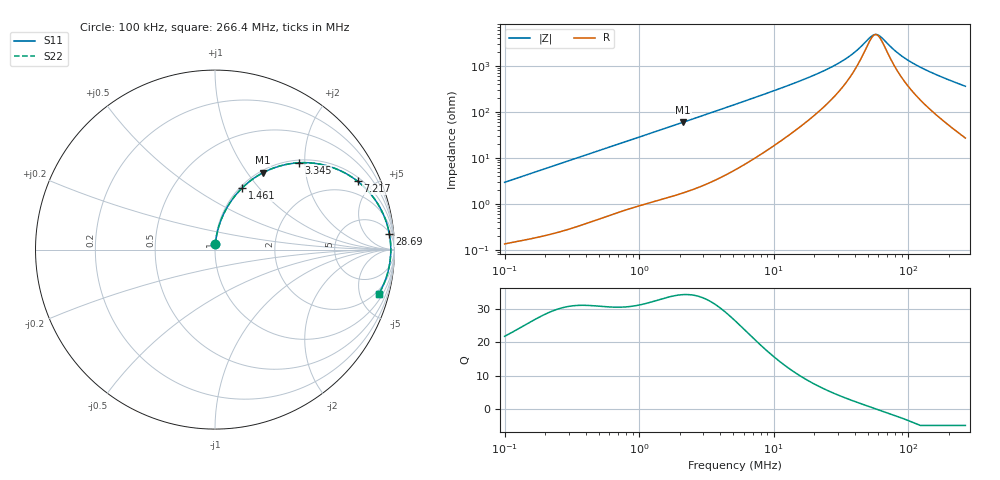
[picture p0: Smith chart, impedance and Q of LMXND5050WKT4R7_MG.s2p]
! LMXND5050WKT4R7_MG  S-PARAMETER MODEL  ( General Type )
! Model Generated by TAIYO YUDEN Corporation (http://www.ty-top.com)
! Version 1.0
! TAIYO YUDEN Control No. 191023NI43SB-FBB
! Copyright(c) 2019 TAIYO YUDEN CO.,LTD. All Rights Reserved.
! Product Description (link to TY-COMPAS)
! https://ds.yuden.co.jp/TYCOMPAS/or/detail?pn=LMXND5050WKT4R7MMG&u=M
! Products Name : Inductors
! Characteristics :
!  Inductance : 4.7 uH , SRF(min) : 37 MHz , DC Resistance(max) : 0.072 Ohm
!  Rated Current : Saturation :2000 mA , Temp Rise : 2000 mA
!  Case Size : 4.9 x 4.9 / 0.193 x 0.193 [mm/inch] , Thickness : 2 / 0.079 [mm/inch]
!  (Conditions: Temperature = 25 degC , DC Bias Current/Voltage = 0A / 0V)
! External Node Assignments :
!  1  o---GGG---o  2
! GND o---------o GND
! Frequency Range : 0.1MHz  -  266.375554MHz  [ 402 STEP ]
# MHz S RI R 50
! Freq[MHz].  S11 Real  S11 Imag  S21 Real  S21 Imag  S12 Real  S12 Imag  S22 Real  S22 Imag
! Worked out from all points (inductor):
!   401 points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, 100 kHz to 266.4 MHz, reference 50 ohm
!   read as one part in series: L = 4.65 uH near 104 kHz
!   highest Q = 34.3 at 2.125 MHz (marker M1), where L = 4.44 uH
!   self-resonance near 57.42 MHz
!   S11 on the Smith chart (normalised r, x): 100 kHz: 1.00, +0.06; 1.461 MHz: 1.02, +0.82; 3.345 MHz: 1.06, +1.87; 7.217 MHz: 1.19, +4.06; 28.69 MHz: 6, +20; 266.4 MHz: 1.54, -7.16
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0.1  0.00221 0.0293  0.9978 -0.0293  0.9978 -0.0293  0.00221 0.0293
0.374775  0.0148 0.1059  0.9852 -0.1059  0.9852 -0.1059  0.0148 0.1059
0.808641  0.0563 0.2147  0.9437 -0.2147  0.9437 -0.2147  0.0563 0.2147
1.404561  0.1419 0.334  0.8581 -0.334  0.8581 -0.334  0.1419 0.334
1.46106  0.1512 0.3434  0.8488 -0.3434  0.8488 -0.3434  0.1512 0.3434
2.125099  0.2665 0.4278  0.7335 -0.4278  0.7335 -0.4278  0.2665 0.4278
3.344606  0.4665 0.4837  0.5335 -0.4837  0.5335 -0.4837  0.4665 0.4837
5.26394  0.6783 0.4484  0.3217 -0.4484  0.3217 -0.4484  0.6783 0.4484
7.216568  0.7941 0.3811  0.2059 -0.3811  0.2059 -0.3811  0.7941 0.3811
11.35786  0.8986 0.268  0.1014 -0.268  0.1014 -0.268  0.8986 0.268
19.34272  0.9543 0.1543  0.0457 -0.1543  0.0457 -0.1543  0.9543 0.1543
28.69407  0.9712 0.0896  0.0288 -0.0896  0.0288 -0.0896  0.9712 0.0896
38.56988  0.977 0.0491  0.023 -0.0491  0.023 -0.0491  0.977 0.0491
51.84469  0.9794 0.0123  0.0206 -0.0123  0.0206 -0.0123  0.9794 0.0123
56.09953  0.9795 0.00279  0.0205 -0.00279  0.0205 -0.00279  0.9795 0.00279
58.35616  0.9795 -0.00196  0.0205 0.00196  0.0205 0.00196  0.9795 -0.00196
61.91244  0.9795 -0.00909  0.0205 0.00909  0.0205 0.00909  0.9795 -0.00909
72.49162  0.9787 -0.0283  0.0213 0.0283  0.0213 0.0283  0.9787 -0.0283
90.05107  0.9764 -0.0559  0.0236 0.0559  0.0236 0.0559  0.9764 -0.0559
118.681  0.9704 -0.0945  0.0296 0.0945  0.0296 0.0945  0.9704 -0.0945
172.6204  0.9538 -0.1568  0.0462 0.1568  0.0462 0.1568  0.9538 -0.1568
266.3756  0.9121 -0.2481  0.0879 0.2481  0.0879 0.2481  0.9121 -0.2481
